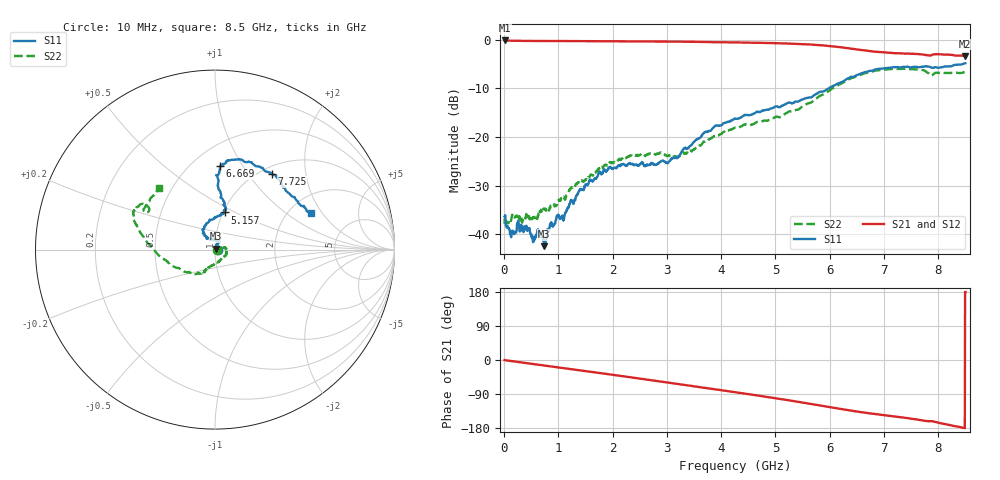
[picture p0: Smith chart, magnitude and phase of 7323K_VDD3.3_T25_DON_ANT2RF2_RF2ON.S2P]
!Agilent Technologies,E5071C,MY46417908,A.11.23
!Date: Mon Jan 18 17:06:21 2021
!Data & Calibration Information:
!Freq	S11:SOLT2(ON)	S21:SOLT2(ON)	S12:SOLT2(ON)	S22:SOLT2(ON)
!PortZ  Port1:50+j0  Port2:50+j0
!Above PortZ is port z conversion or system Z0 setting when saving the data.
!When reading, reference impedance value at option line is always used.
# Hz S dB R 50
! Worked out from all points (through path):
!   1601 points, 10 MHz to 8.5 GHz, reference 50 ohm
!   highest |S21| = -0.16 dB at 10 MHz (marker M1); lowest = -3.4 dB at 8.495 GHz (marker M2)
!   group delay of S21, straight-line fit = 58.4 ps
!   lowest |S11| = -42.5 dB at 742.3 MHz (marker M3), VSWR 1.02, Z = 50.6 + j0.437 ohm
!   |S11| at or under -10 dB: start of sweep to 5.983 GHz
!   |S22| runs from -37.9 to -6.0 dB; largest |S21 - S12| = 0.0084
!   S11 on the Smith chart (normalised r, x): 10 MHz: 1.03, +0.00; 5.157 GHz: 1.02, +0.44; 6.669 GHz: 0.67, +0.80; 7.725 GHz: 1.12, +1.30; 8.5 GHz: 2.60, +1.58
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1e7  -36.36 0.0  -0.16 -0.3  -0.16 -0.3  -37.89 -11.0
1.479625e8  -39.31 1.5  -0.21 -3.1  -0.21 -3.1  -36.02 -2.5
2.85925e8  -39.37 -4.7  -0.23 -5.8  -0.23 -5.8  -36.69 -5.1
5.724625e8  -40.90 7.9  -0.27 -11.3  -0.27 -11.3  -36.63 -10.6
6.4675e8  -39.90 16.2  -0.27 -12.7  -0.26 -12.7  -35.96 -2.3
7.422625e8  -42.47 35.0  -0.27 -14.6  -0.27 -14.6  -34.95 -2.7
8.430812e8  -38.24 44.1  -0.28 -16.5  -0.28 -16.5  -34.49 4.3
1.103088e9  -36.89 66.9  -0.28 -21.6  -0.29 -21.5  -32.32 2.5
1.426769e9  -30.85 72.1  -0.30 -27.8  -0.30 -27.9  -28.99 12.7
1.946781e9  -26.17 64.0  -0.32 -38.0  -0.32 -38.0  -25.23 12.9
2.843538e9  -25.50 88.0  -0.37 -56.0  -0.37 -56.0  -23.50 -26.2
3.204362e9  -24.18 114.7  -0.39 -63.4  -0.39 -63.4  -24.10 -57.5
3.692538e9  -19.04 125.4  -0.47 -73.5  -0.47 -73.5  -21.01 -100.2
4.255e9  -16.21 107.7  -0.57 -84.9  -0.57 -85.0  -18.13 -114.7
5.157062e9  -13.40 75.4  -0.75 -104.3  -0.75 -104.4  -15.37 -127.1
5.671769e9  -11.79 78.5  -1.01 -116.2  -1.00 -116.3  -12.81 -153.4
6.669344e9  -6.63 86.4  -2.24 -139.4  -2.26 -139.4  -6.85 163.0
7.088538e9  -5.77 77.6  -2.69 -147.1  -2.70 -147.3  -6.06 156.4
7.725288e9  -5.58 53.1  -3.07 -160.0  -3.09 -160.0  -6.25 148.8
7.916312e9  -5.77 42.0  -3.03 -162.5  -3.04 -162.6  -7.04 151.8
8.494694e9  -4.86 21.1  -3.36 179.8  -3.45 179.5  -6.65 132.7
8.5e9  -4.84 21.0  -3.36 179.6  -3.44 179.3  -6.64 132.2
